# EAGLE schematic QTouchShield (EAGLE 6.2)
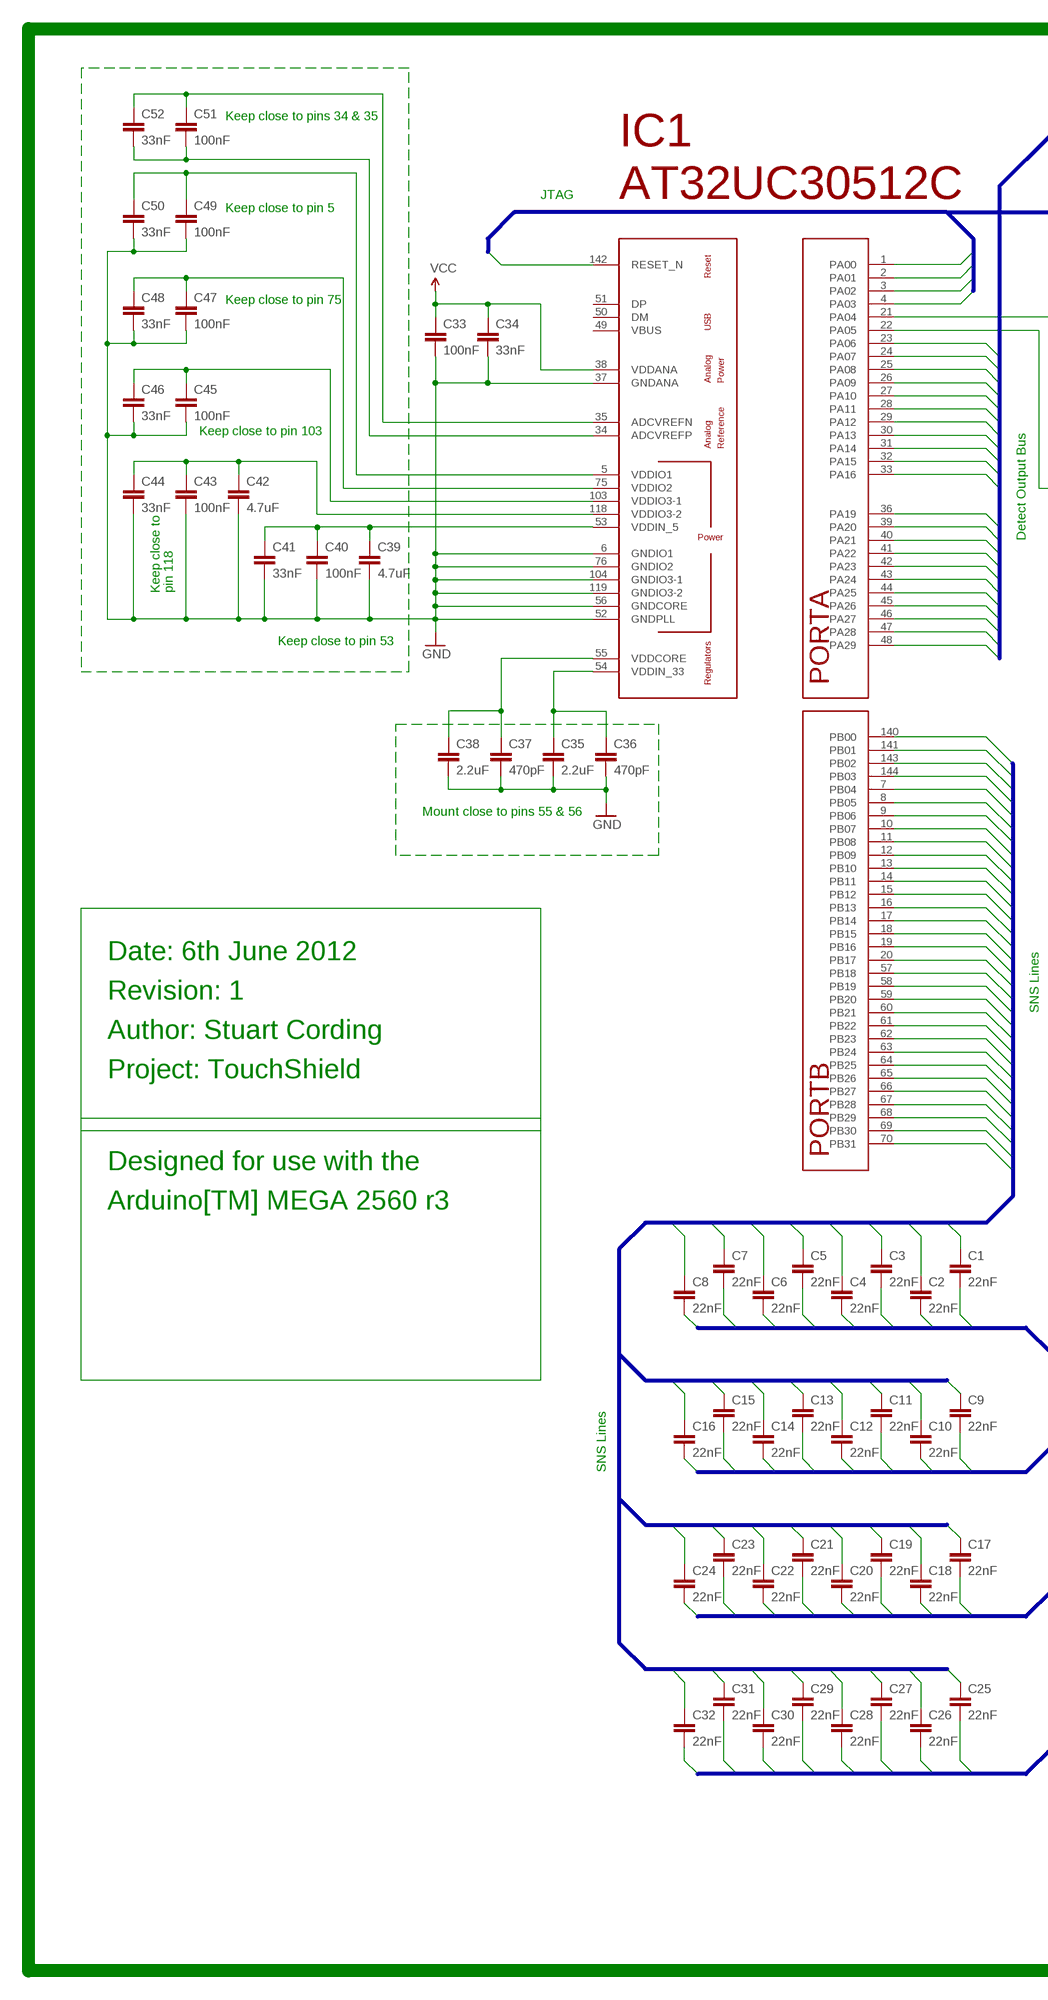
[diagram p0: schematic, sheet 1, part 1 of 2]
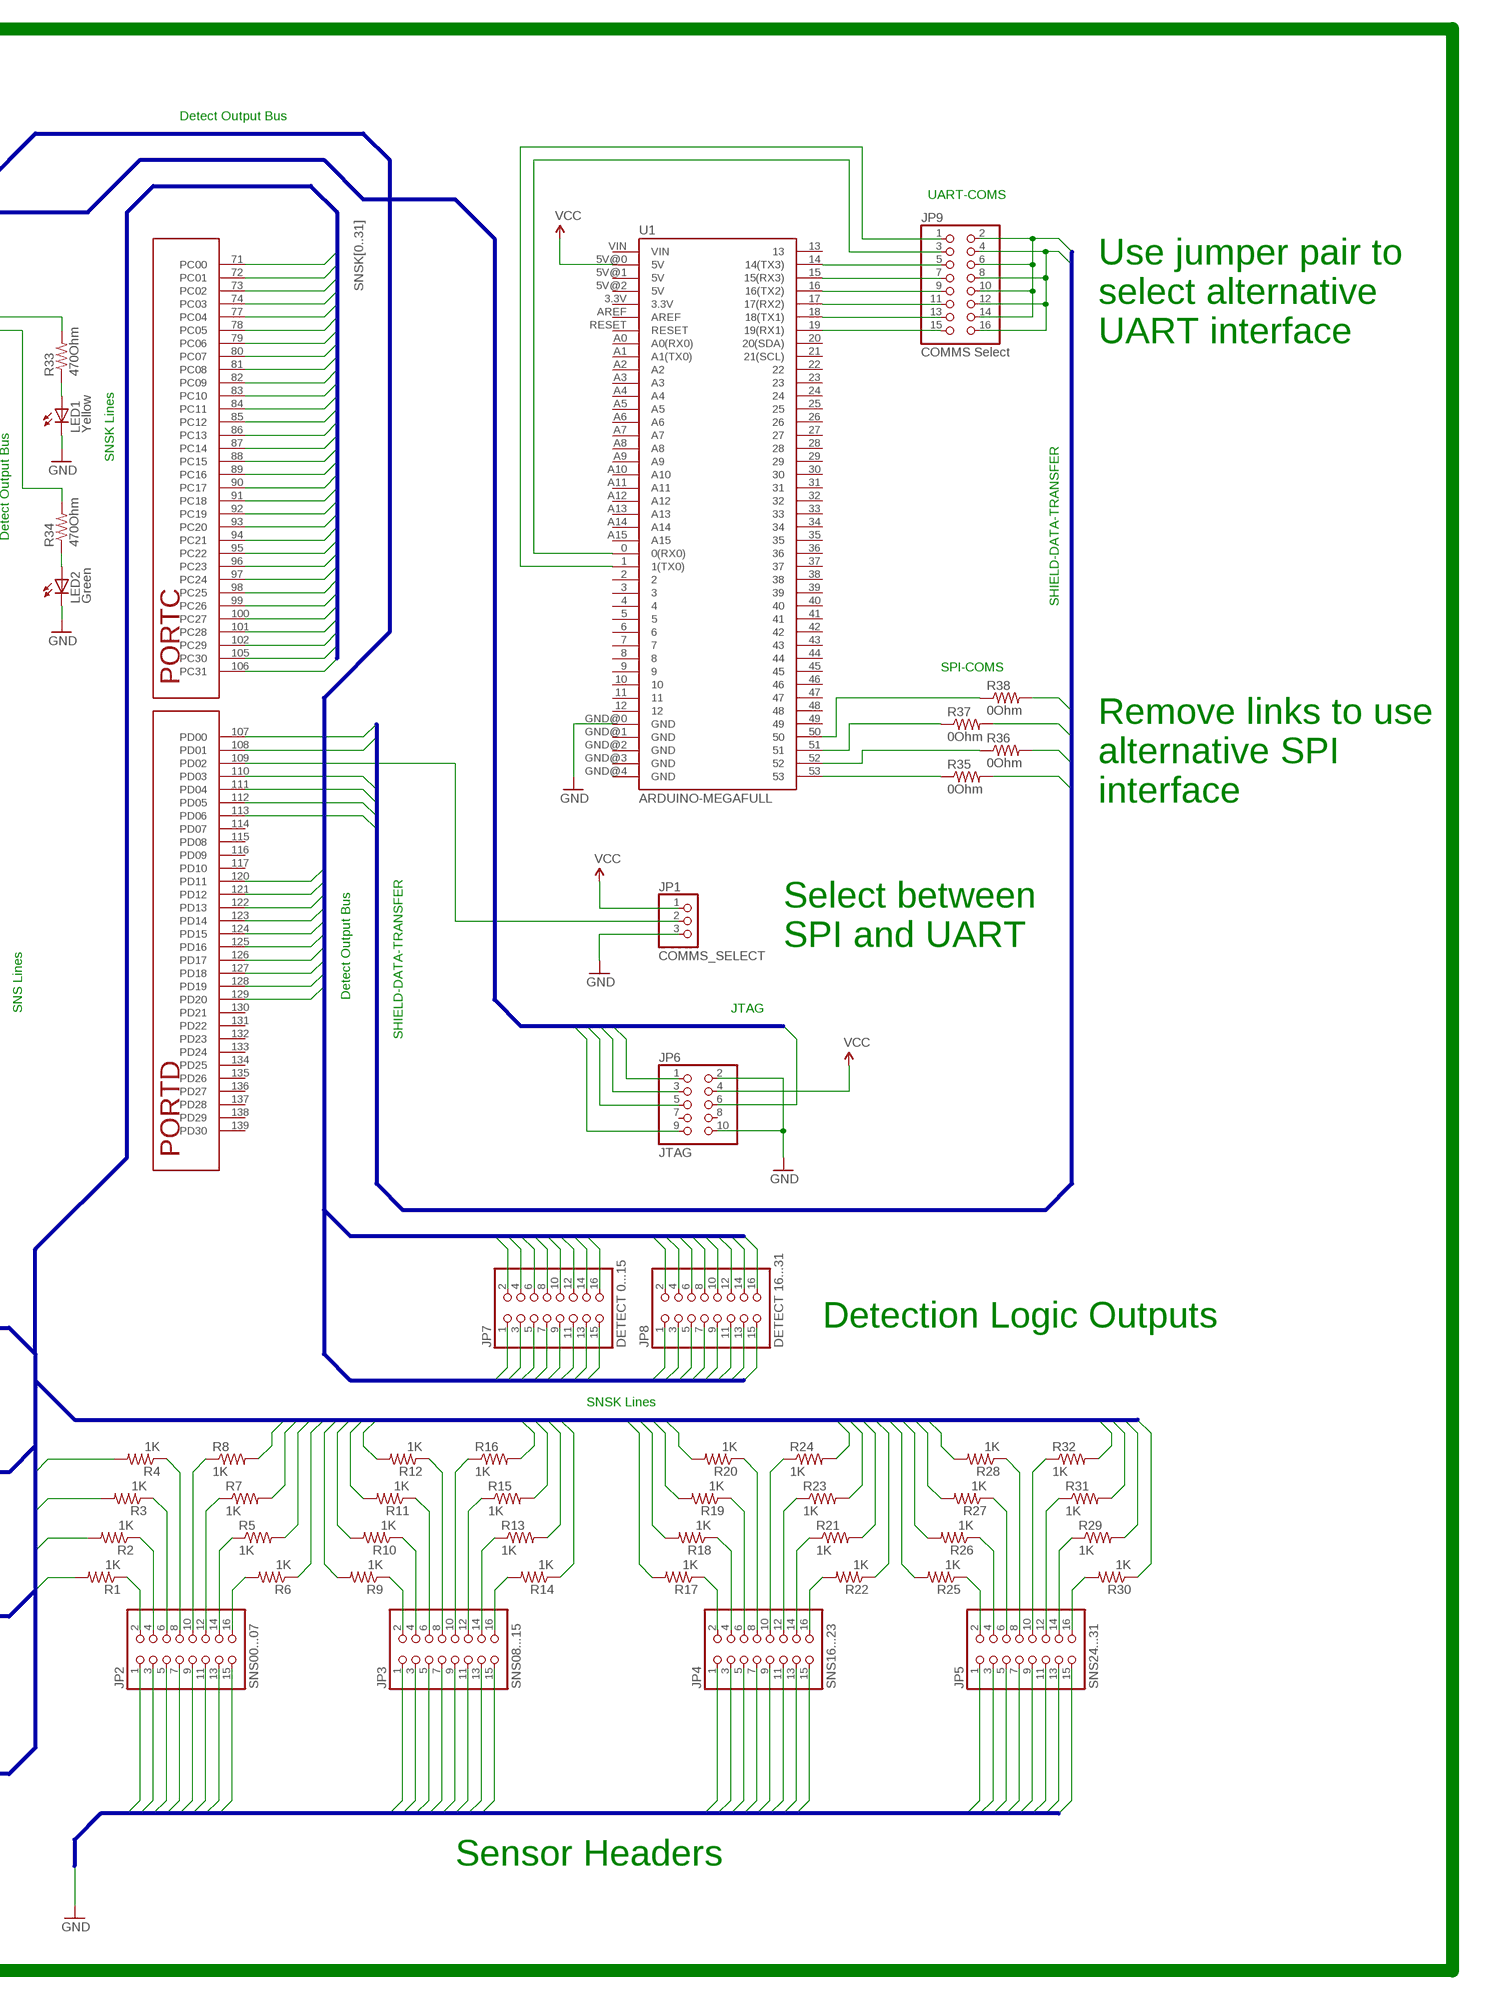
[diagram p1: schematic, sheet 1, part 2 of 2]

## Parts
C1  22nF  CAP0805  [0805]
C2  22nF  CAP0805  [0805]
C3  22nF  CAP0805  [0805]
C4  22nF  CAP0805  [0805]
C5  22nF  CAP0805  [0805]
C6  22nF  CAP0805  [0805]
C7  22nF  CAP0805  [0805]
C8  22nF  CAP0805  [0805]
C9  22nF  CAP0805  [0805]
C10  22nF  CAP0805  [0805]
C11  22nF  CAP0805  [0805]
C12  22nF  CAP0805  [0805]
C13  22nF  CAP0805  [0805]
C14  22nF  CAP0805  [0805]
C15  22nF  CAP0805  [0805]
C16  22nF  CAP0805  [0805]
C17  22nF  CAP0805  [0805]
C18  22nF  CAP0805  [0805]
C19  22nF  CAP0805  [0805]
C20  22nF  CAP0805  [0805]
C21  22nF  CAP0805  [0805]
C22  22nF  CAP0805  [0805]
C23  22nF  CAP0805  [0805]
C24  22nF  CAP0805  [0805]
C25  22nF  CAP0805  [0805]
C26  22nF  CAP0805  [0805]
C27  22nF  CAP0805  [0805]
C28  22nF  CAP0805  [0805]
C29  22nF  CAP0805  [0805]
C30  22nF  CAP0805  [0805]
C31  22nF  CAP0805  [0805]
C32  22nF  CAP0805  [0805]
C33  100nF  CAP0805  [0805]
C34  33nF  CAP0805  [0805]
C35  2.2uF  CAP1210  [1210]
C36  470pF  CAP0805  [0805]
C37  470pF  CAP0805  [0805]
C38  2.2uF  CAP1210  [1210]
C39  4.7uF  CAP1210  [1210]
C40  100nF  CAP0805  [0805]
C41  33nF  CAP0805  [0805]
C42  4.7uF  CAP1210  [1210]
C43  100nF  CAP0805  [0805]
C44  33nF  CAP0805  [0805]
C45  100nF  CAP0805  [0805]
C46  33nF  CAP0805  [0805]
C47  100nF  CAP0805  [0805]
C48  33nF  CAP0805  [0805]
C49  100nF  CAP0805  [0805]
C50  33nF  CAP0805  [0805]
C51  100nF  CAP0805  [0805]
C52  33nF  CAP0805  [0805]
IC1  AT32UC3C0512C  [LQFP144]
JP1  COMMS_SELECT  PINHD-1X3  [1X03]
JP2  SNS00...07  PINHD-2X8  [2X08]
JP3  SNS08...15  PINHD-2X8  [2X08]
JP4  SNS16...23  PINHD-2X8  [2X08]
JP5  SNS24...31  PINHD-2X8  [2X08]
JP6  JTAG  PINHD-2X5  [2X05]
JP7  DETECT 0...15  PINHD-2X8  [2X08]
JP8  DETECT 16...31  PINHD-2X8  [2X08]
JP9  COMMS Select  PINHD-2X8  [2X08]
LED1  Yellow  LED1206  [LED-1206]
LED2  Green  LED1206  [LED-1206]
R1  1K  RESISTOR0805-RES  [0805]
R2  1K  RESISTOR0805-RES  [0805]
R3  1K  RESISTOR0805-RES  [0805]
R4  1K  RESISTOR0805-RES  [0805]
R5  1K  RESISTOR0805-RES  [0805]
R6  1K  RESISTOR0805-RES  [0805]
R7  1K  RESISTOR0805-RES  [0805]
R8  1K  RESISTOR0805-RES  [0805]
R9  1K  RESISTOR0805-RES  [0805]
R10  1K  RESISTOR0805-RES  [0805]
R11  1K  RESISTOR0805-RES  [0805]
R12  1K  RESISTOR0805-RES  [0805]
R13  1K  RESISTOR0805-RES  [0805]
R14  1K  RESISTOR0805-RES  [0805]
R15  1K  RESISTOR0805-RES  [0805]
R16  1K  RESISTOR0805-RES  [0805]
R17  1K  RESISTOR0805-RES  [0805]
R18  1K  RESISTOR0805-RES  [0805]
R19  1K  RESISTOR0805-RES  [0805]
R20  1K  RESISTOR0805-RES  [0805]
R21  1K  RESISTOR0805-RES  [0805]
R22  1K  RESISTOR0805-RES  [0805]
R23  1K  RESISTOR0805-RES  [0805]
R24  1K  RESISTOR0805-RES  [0805]
R25  1K  RESISTOR0805-RES  [0805]
R26  1K  RESISTOR0805-RES  [0805]
R27  1K  RESISTOR0805-RES  [0805]
R28  1K  RESISTOR0805-RES  [0805]
R29  1K  RESISTOR0805-RES  [0805]
R30  1K  RESISTOR0805-RES  [0805]
R31  1K  RESISTOR0805-RES  [0805]
R32  1K  RESISTOR0805-RES  [0805]
R33  470Ohm  RESISTOR0805-RES  [0805]
R34  470Ohm  RESISTOR0805-RES  [0805]
R35  0Ohm  RESISTOR0805-RES  [0805]
R36  0Ohm  RESISTOR0805-RES  [0805]
R37  0Ohm  RESISTOR0805-RES  [0805]
R38  0Ohm  RESISTOR0805-RES  [0805]
U1  ARDUINO-MEGAFULL  [ARDUINO_MEGA]

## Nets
ADCVREFN: C51.1 C52.1 IC1.35(ADCVREFN)
ADCVREFP: C51.2 C52.2 IC1.34(ADCVREFP)
GND: C33.2 C34.2 C35.2 C36.2 C37.2 C38.2 C39.2 C40.2 C41.2 C42.2 C43.2 C44.2 C45.2 C46.2 C47.2 C48.2 C49.2 C50.2 IC1.6(GNDIO1) IC1.37(GNDANA) IC1.52(GNDPLL) IC1.56(GNDCORE) IC1.76(GNDIO2) IC1.104(GNDIO3-1) IC1.119(GNDIO3-2) JP1.3 JP2.1 JP2.3 JP2.5 JP2.7 JP2.9 JP2.11 JP2.13 JP2.15 JP3.1 JP3.3 JP3.5 JP3.7 JP3.9 JP3.11 JP3.13 JP3.15 JP4.1 JP4.3 JP4.5 JP4.7 JP4.9 JP4.11 JP4.13 JP4.15 JP5.1 JP5.3 JP5.5 JP5.7 JP5.9 JP5.11 JP5.13 JP5.15 JP6.2 JP6.10 LED1.C LED2.C U1.GND@0(GND)
JTAG_RESET: IC1.142(RESET_N) JP6.6
JTAG_TCK: IC1.1(PA00) JP6.1
JTAG_TDI: IC1.2(PA01) JP6.9
JTAG_TDO: IC1.3(PA02) JP6.3
JTAG_TMS: IC1.4(PA03) JP6.5
MISO-PIN50: R38.1 U1.50
MOSI-PIN51: R37.1 U1.51
N$1: LED1.A R33.1
N$2: JP2.2 R1.1
N$3: JP2.4 R2.1
N$4: JP2.6 R3.1
N$5: JP2.8 R4.1
N$6: JP2.10 R8.1
N$7: JP2.12 R7.1
N$8: JP2.14 R5.1
N$9: JP2.16 R6.2
N$10: JP3.2 R9.1
N$11: JP3.4 R10.1
N$12: JP3.6 R11.1
N$13: JP3.8 R12.1
N$14: JP3.10 R16.1
N$15: JP3.12 R15.1
N$16: JP3.14 R13.1
N$17: JP3.16 R14.2
N$18: JP4.2 R17.1
N$19: JP4.4 R18.1
N$20: JP4.6 R19.1
N$21: JP4.8 R20.1
N$22: JP4.10 R24.1
N$23: JP4.12 R23.1
N$24: JP4.14 R21.1
N$25: JP4.16 R22.2
N$26: JP5.2 R25.1
N$27: JP5.4 R26.1
N$28: JP5.6 R27.1
N$29: JP5.8 R28.1
N$30: JP5.10 R32.1
N$31: JP5.12 R31.1
N$32: JP5.14 R29.1
N$33: JP5.16 R30.2
N$42: LED2.A R34.1
QT-DETECT-GENERAL: IC1.21(PA04) R33.2
RX0: JP9.3 U1.0(0(RX0))
RX1: JP9.15 U1.19(19(RX1))
RX2: JP9.11 U1.17(17(RX2))
RX3: JP9.7 U1.15(15(RX3))
SCK-PIN52: R36.1 U1.52
SDT-SPI0-MISO: IC1.112(PD05) R37.2
SDT-SPI0-MOSI: IC1.111(PD04) R38.2
SDT-SPI0-SCK: IC1.113(PD06) R36.2
SDT-SPI0-SS: IC1.110(PD03) R35.2
SDT-USART0-RXD: IC1.108(PD01) JP9.4 JP9.8 JP9.12 JP9.16
SDT-USART0-TXD: IC1.107(PD00) JP9.2 JP9.6 JP9.10 JP9.14
SHIELD-DATA-TRANSFER-COM-SELECT: IC1.109(PD02) JP1.2
SHIELD-DATA-TRANSFER-VISUAL-OUTPUT: IC1.22(PA05) R34.2
SHIELD-DETECT0: IC1.23(PA06) JP7.1
SHIELD-DETECT1: IC1.24(PA07) JP7.2
SHIELD-DETECT2: IC1.25(PA08) JP7.3
SHIELD-DETECT3: IC1.26(PA09) JP7.4
SHIELD-DETECT4: IC1.27(PA10) JP7.5
SHIELD-DETECT5: IC1.28(PA11) JP7.6
SHIELD-DETECT6: IC1.29(PA12) JP7.7
SHIELD-DETECT7: IC1.30(PA13) JP7.8
SHIELD-DETECT8: IC1.31(PA14) JP7.9
SHIELD-DETECT9: IC1.32(PA15) JP7.10
SHIELD-DETECT10: IC1.33(PA16) JP7.11
SHIELD-DETECT11: IC1.36(PA19) JP7.12
SHIELD-DETECT12: IC1.39(PA20) JP7.13
SHIELD-DETECT13: IC1.40(PA21) JP7.14
SHIELD-DETECT14: IC1.41(PA22) JP7.15
SHIELD-DETECT15: IC1.42(PA23) JP7.16
SHIELD-DETECT16: IC1.43(PA24) JP8.1
SHIELD-DETECT17: IC1.44(PA25) JP8.2
SHIELD-DETECT18: IC1.45(PA26) JP8.3
SHIELD-DETECT19: IC1.46(PA27) JP8.4
SHIELD-DETECT20: IC1.47(PA28) JP8.5
SHIELD-DETECT21: IC1.48(PA29) JP8.6
SHIELD-DETECT22: IC1.120(PD11) JP8.7
SHIELD-DETECT23: IC1.121(PD12) JP8.8
SHIELD-DETECT24: IC1.122(PD13) JP8.9
SHIELD-DETECT25: IC1.123(PD14) JP8.10
SHIELD-DETECT26: IC1.124(PD15) JP8.11
SHIELD-DETECT27: IC1.125(PD16) JP8.12
SHIELD-DETECT28: IC1.126(PD17) JP8.13
SHIELD-DETECT29: IC1.127(PD18) JP8.14
SHIELD-DETECT30: IC1.128(PD19) JP8.15
SHIELD-DETECT31: IC1.129(PD20) JP8.16
SNS0: C1.1 IC1.140(PB00)
SNS1: C2.1 IC1.141(PB01)
SNS2: C3.1 IC1.143(PB02)
SNS3: C4.1 IC1.144(PB03)
SNS4: C5.1 IC1.7(PB04)
SNS5: C6.1 IC1.8(PB05)
SNS6: C7.1 IC1.9(PB06)
SNS7: C8.1 IC1.10(PB07)
SNS8: C9.1 IC1.11(PB08)
SNS9: C10.1 IC1.12(PB09)
SNS10: C11.1 IC1.13(PB10)
SNS11: C12.1 IC1.14(PB11)
SNS12: C13.1 IC1.15(PB12)
SNS13: C14.1 IC1.16(PB13)
SNS14: C15.1 IC1.17(PB14)
SNS15: C16.1 IC1.18(PB15)
SNS16: C17.1 IC1.19(PB16)
SNS17: C18.1 IC1.20(PB17)
SNS18: C19.1 IC1.57(PB18)
SNS19: C20.1 IC1.58(PB19)
SNS20: C21.1 IC1.59(PB20)
SNS21: C22.1 IC1.60(PB21)
SNS22: C23.1 IC1.61(PB22)
SNS23: C24.1 IC1.62(PB23)
SNS24: C25.1 IC1.63(PB24)
SNS25: C26.1 IC1.64(PB25)
SNS26: C27.1 IC1.65(PB26)
SNS27: C28.1 IC1.66(PB27)
SNS28: C29.1 IC1.67(PB28)
SNS29: C30.1 IC1.68(PB29)
SNS30: C31.1 IC1.69(PB30)
SNS31: C32.1 IC1.70(PB31)
SNSK0: C1.2 IC1.71(PC00) R1.2
SNSK1: C2.2 IC1.72(PC01) R2.2
SNSK2: C3.2 IC1.73(PC02) R3.2
SNSK3: C4.2 IC1.74(PC03) R4.2
SNSK4: C5.2 IC1.77(PC04) R8.2
SNSK5: C6.2 IC1.78(PC05) R7.2
SNSK6: C7.2 IC1.79(PC06) R5.2
SNSK7: C8.2 IC1.80(PC07) R6.1
SNSK8: C9.2 IC1.81(PC08) R9.2
SNSK9: C10.2 IC1.82(PC09) R10.2
SNSK10: C11.2 IC1.83(PC10) R11.2
SNSK11: C12.2 IC1.84(PC11) R12.2
SNSK12: C13.2 IC1.85(PC12) R16.2
SNSK13: C14.2 IC1.86(PC13) R15.2
SNSK14: C15.2 IC1.87(PC14) R13.2
SNSK15: C16.2 IC1.88(PC15) R14.1
SNSK16: C17.2 IC1.89(PC16) R17.2
SNSK17: C18.2 IC1.90(PC17) R18.2
SNSK18: C19.2 IC1.91(PC18) R19.2
SNSK19: C20.2 IC1.92(PC19) R20.2
SNSK20: C21.2 IC1.93(PC20) R24.2
SNSK21: C22.2 IC1.94(PC21) R23.2
SNSK22: C23.2 IC1.95(PC22) R21.2
SNSK23: C24.2 IC1.96(PC23) R22.1
SNSK24: C25.2 IC1.97(PC24) R25.2
SNSK25: C26.2 IC1.98(PC25) R26.2
SNSK26: C27.2 IC1.99(PC26) R27.2
SNSK27: C28.2 IC1.100(PC27) R28.2
SNSK28: C29.2 IC1.101(PC28) R32.2
SNSK29: C30.2 IC1.102(PC29) R31.2
SNSK30: C31.2 IC1.105(PC30) R29.2
SNSK31: C32.2 IC1.106(PC31) R30.1
SS-PIN53: R35.1 U1.53
TX0: JP9.1 U1.1(1(TX0))
TX1: JP9.13 U1.18(18(TX1))
TX2: JP9.9 U1.16(16(TX2))
TX3: JP9.5 U1.14(14(TX3))
VCC: C33.1 C34.1 IC1.38(VDDANA) JP1.1 JP6.4 U1.5V@0(5V)
VDDCORE: C37.1 C38.1 IC1.55(VDDCORE)
VDDIN_5: C39.1 C40.1 C41.1 IC1.53(VDDIN_5)
VDDIN_33: C35.1 C36.1 IC1.54(VDDIN_33)
VDDIO1: C49.1 C50.1 IC1.5(VDDIO1)
VDDIO2: C47.1 C48.1 IC1.75(VDDIO2)
VDDIO3_1: C45.1 C46.1 IC1.103(VDDIO3-1)
VDDIO3_2: C42.1 C43.1 C44.1 IC1.118(VDDIO3-2)
Unconnected: IC1.49(VBUS) IC1.50(DM) IC1.51(DP) IC1.114(PD07) IC1.115(PD08) IC1.116(PD09) IC1.117(PD10) IC1.130(PD21) IC1.131(PD22) IC1.132(PD23) IC1.133(PD24) IC1.134(PD25) IC1.135(PD26) IC1.136(PD27) IC1.137(PD28) IC1.138(PD29) IC1.139(PD30) JP6.7 JP6.8 U1.2 U1.3 U1.3.3V U1.4 U1.5 U1.5V@1(5V) U1.5V@2(5V) U1.6 U1.7 U1.8 U1.9 U1.10 U1.11 U1.12 U1.13 U1.20(20(SDA)) U1.21(21(SCL)) U1.22 U1.23 U1.24 U1.25 U1.26 U1.27 U1.28 U1.29 U1.30 U1.31 U1.32 U1.33 U1.34 U1.35 U1.36 U1.37 U1.38 U1.39 U1.40 U1.41 U1.42 U1.43 U1.44 U1.45 U1.46 U1.47 U1.48 U1.49 U1.A0(A0(RX0)) U1.A1(A1(TX0)) U1.A2 U1.A3 U1.A4 U1.A5 U1.A6 U1.A7 U1.A8 U1.A9 U1.A10 U1.A11 U1.A12 U1.A13 U1.A14 U1.A15 U1.AREF U1.GND@1(GND) U1.GND@2(GND) U1.GND@3(GND) U1.GND@4(GND) U1.RESET U1.VIN

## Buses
SNS[0..31]
SNSK[0..31]
GND
JTAG_TCK,JTAG_TDI,JTAG_TDO,JTAG_TMS,JTAG_RESET
SHIELD-DETECT[0..31]
SDT-USART0-TXD,SDT-USART0-RXD,SDT-SPI0-SS,SDT-SPI0-MOSI,SDT-SPI0-MISO,SDT-SPI0-SCK

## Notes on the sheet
- Keep close to pins 34 & 35 | Detect Output Bus
- JTAG | UART-COMS
- Keep close to pin 5
- Use jumper pair to
- Keep close to pin 75 | select alternative
- UART interface
- Keep close to pin 103
- SNSK Lines
- Detect Output Bus
- Keep close to | pin 118
- SHIELD-DATA-TRANSFER
- Keep close to pin 53
- SPI-COMS
- Remove links to use
- alternative SPI
- interface
- Mount close to pins 55 & 56
- Select between
- SPI and UART
- Date: 6th June 2012
- Revision: 1 | Detect Output Bus
- SNS Lines | JTAG
- Author: Stuart Cording | SHIELD-DATA-TRANSFER
- Project: TouchShield
- Designed for use with the
- Arduino[TM] MEGA 2560 r3
- Detection Logic Outputs
- SNSK Lines
- SNS Lines
- Sensor Headers

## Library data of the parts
C1-C52 = SparkFun:CAP: Capacitor
IC1 = atmel-AVR32:AT32UC3C0512C
JP1 = pinhead:PINHD-1X3: PIN HEADER
JP2-JP5 JP7-JP9 = pinhead:PINHD-2X8: PIN HEADER
JP6 = pinhead:PINHD-2X5: PIN HEADER
LED1 LED2 = SparkFun:LED: LEDs
R1-R38 = SparkFun:RESISTOR: Resistor
U1 = SparkFun:ARDUINO-MEGA: Arduino Mega footprint connections

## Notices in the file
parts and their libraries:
SparkFun: Licensing: CC v3.0 Share-Alike You are welcome to use this library for commercial purposes.
